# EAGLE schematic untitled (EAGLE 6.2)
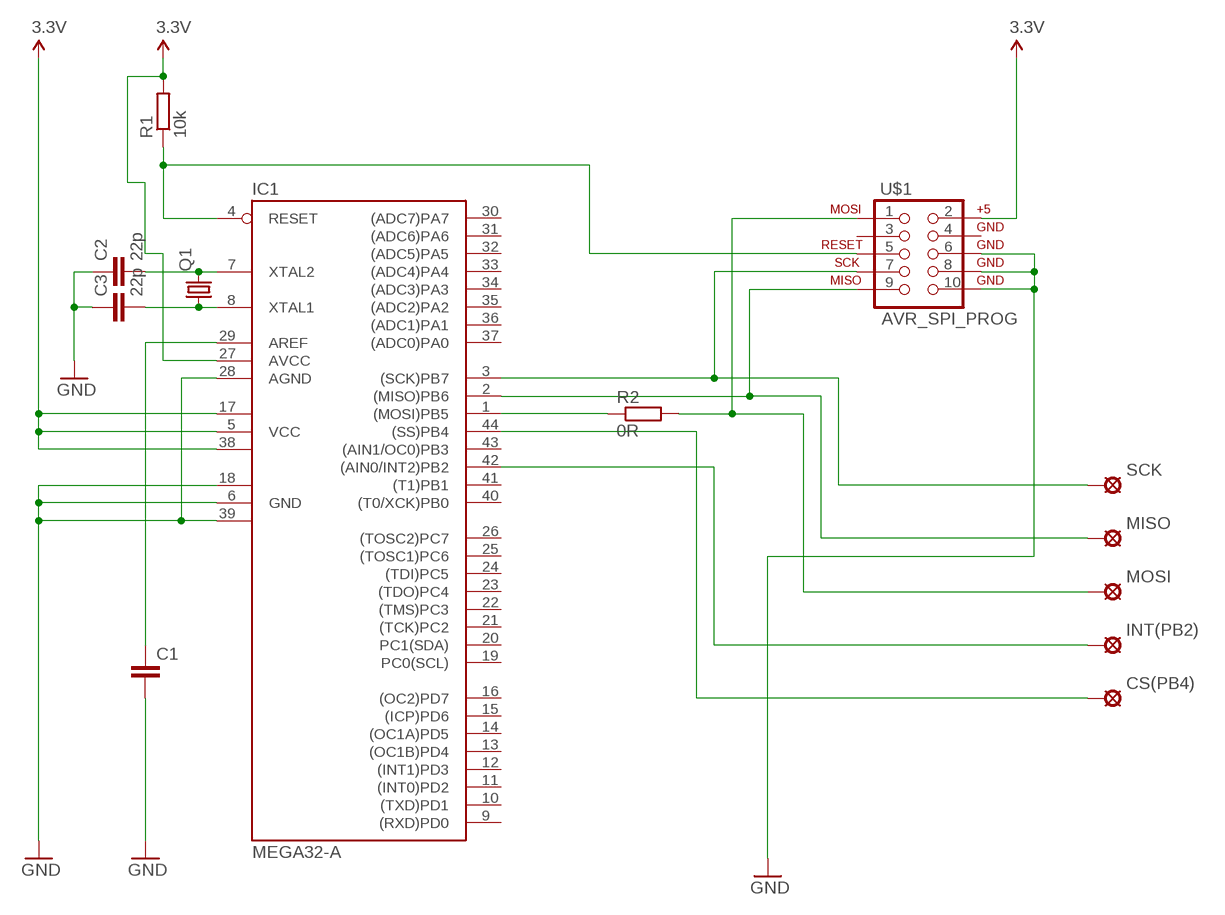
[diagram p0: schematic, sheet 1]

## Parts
C1  C-EUC2220K  [C2220K]
C2  22p  C-EUC1206K  [C1206K]
C3  22p  C-EUC1206K  [C1206K]
CS(PB4)  MCS08  [MCS08]
IC1  MEGA32-A  [TQFP44]
INT(PB2)  MCS08  [MCS08]
MISO  MCS08  [MCS08]
MOSI  MCS08  [MCS08]
Q1  CRYSTALHC49U-V  [HC49U-V]
R1  10k  R-EU_M1206  [M1206]
R2  0R  R-EU_R1206  [R1206]
SCK  MCS08  [MCS08]
U$1  AVR_SPI_PROG  [AVR_ICSP]

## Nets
3.3V: IC1.5(VCC) IC1.17(VCC1) IC1.27(AVCC) IC1.38(VCC2) R1.2 U$1.2
GND: C1.2 C2.1 C3.1 IC1.6(GND) IC1.18(GND1) IC1.28(AGND) IC1.39(GND2) U$1.6 U$1.8 U$1.10
N$1: IC1.42((AIN0/INT2)PB2) INT(PB2).MP
N$2: CS(PB4).MP IC1.44((SS)PB4)
N$3: C1.1 IC1.29(AREF)
N$4: C2.2 IC1.7(XTAL2) Q1.2
N$5: C3.2 IC1.8(XTAL1) Q1.1
N$6: IC1.4(RESET) R1.1 U$1.5
N$7: IC1.1((MOSI)PB5) R2.1
N$8: MOSI.MP R2.2 U$1.1
N$10: IC1.3((SCK)PB7) SCK.MP U$1.7
N$11: IC1.2((MISO)PB6) MISO.MP U$1.9
Unconnected: IC1.9((RXD)PD0) IC1.10((TXD)PD1) IC1.11((INT0)PD2) IC1.12((INT1)PD3) IC1.13((OC1B)PD4) IC1.14((OC1A)PD5) IC1.15((ICP)PD6) IC1.16((OC2)PD7) IC1.19(PC0(SCL)) IC1.20(PC1(SDA)) IC1.21((TCK)PC2) IC1.22((TMS)PC3) IC1.23((TDO)PC4) IC1.24((TDI)PC5) IC1.25((TOSC1)PC6) IC1.26((TOSC2)PC7) IC1.30((ADC7)PA7) IC1.31((ADC6)PA6) IC1.32((ADC5)PA5) IC1.33((ADC4)PA4) IC1.34((ADC3)PA3) IC1.35((ADC2)PA2) IC1.36((ADC1)PA1) IC1.37((ADC0)PA0) IC1.40((T0/XCK)PB0) IC1.41((T1)PB1) IC1.43((AIN1/OC0)PB3) U$1.3 U$1.4

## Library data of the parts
C1-C3 = rcl:C-EU: CAPACITOR, European symbol
CS(PB4) INT(PB2) MISO MOSI SCK = solpad:MCS08: SOLDER PAD
IC1 = avr-7:MEGA32: MICROCONTROLLER 32 Kbytes FLASH 2 Kbytes SRAM 1 Kbytes EEPROM USART 8-channel 10 bit ADC
Q1 = crystal:CRYSTAL: CRYSTAL; OC_FARNELL: 1666969; OC_NEWARK: unknown
R1 R2 = rcl:R-EU_: RESISTOR, European symbol
U$1 = SparkFun:AVR_SPI_PROG: AVR ICSP Header This is the standard AVR In Circuit Serial Programming header. Minimal, but includes pin one indicator. Works with standard Olimex programmers. Also look for the 6-pin reduced version. Spark Fun Electronics SKU: PRT-00778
